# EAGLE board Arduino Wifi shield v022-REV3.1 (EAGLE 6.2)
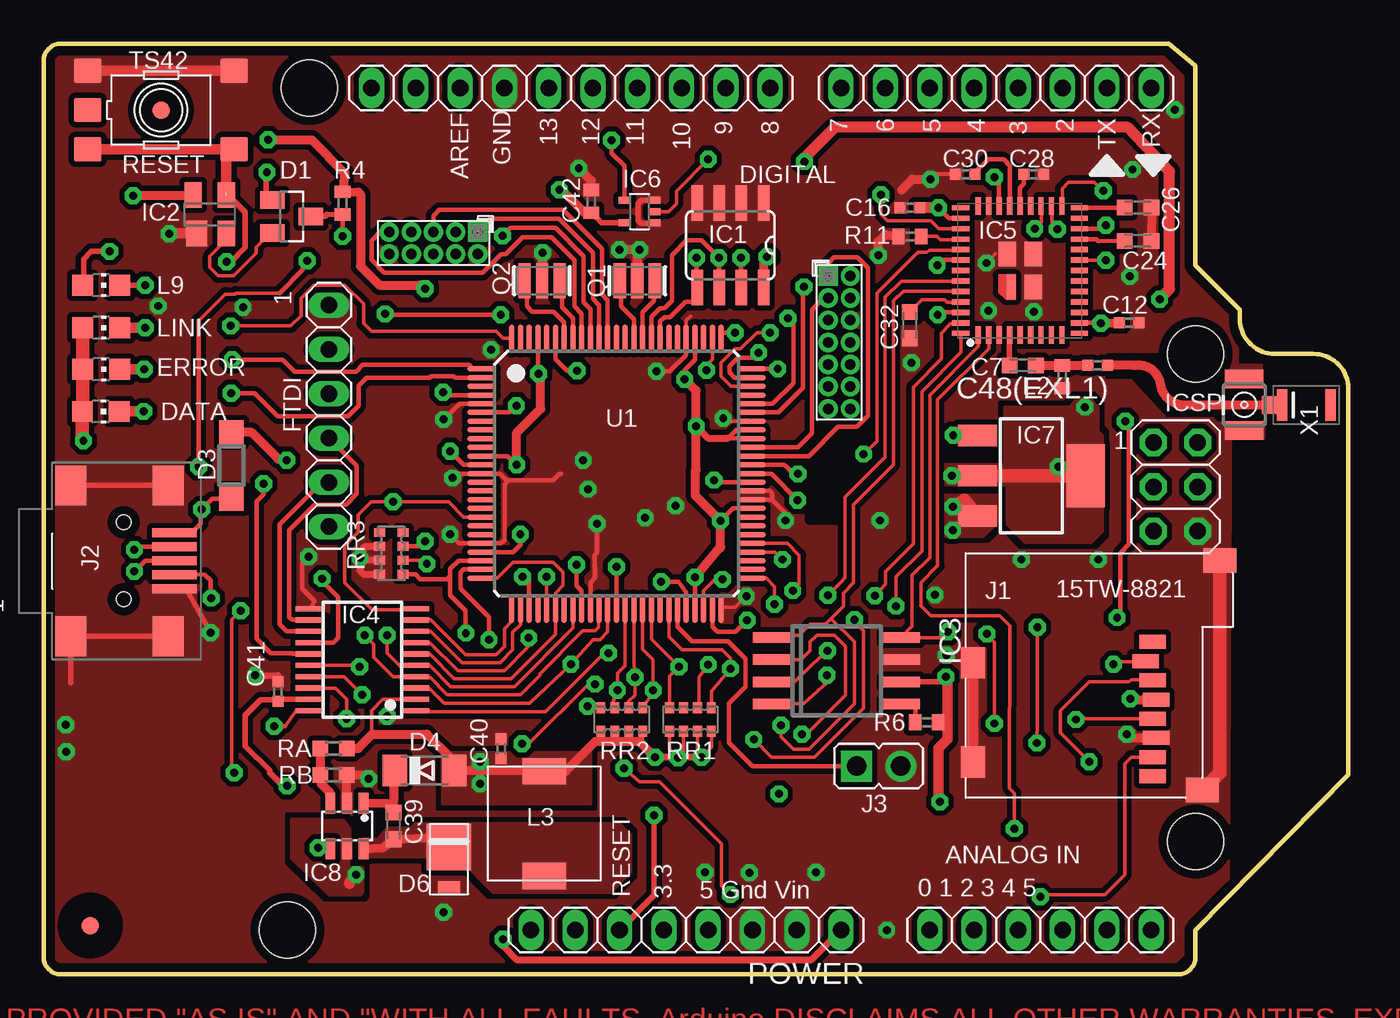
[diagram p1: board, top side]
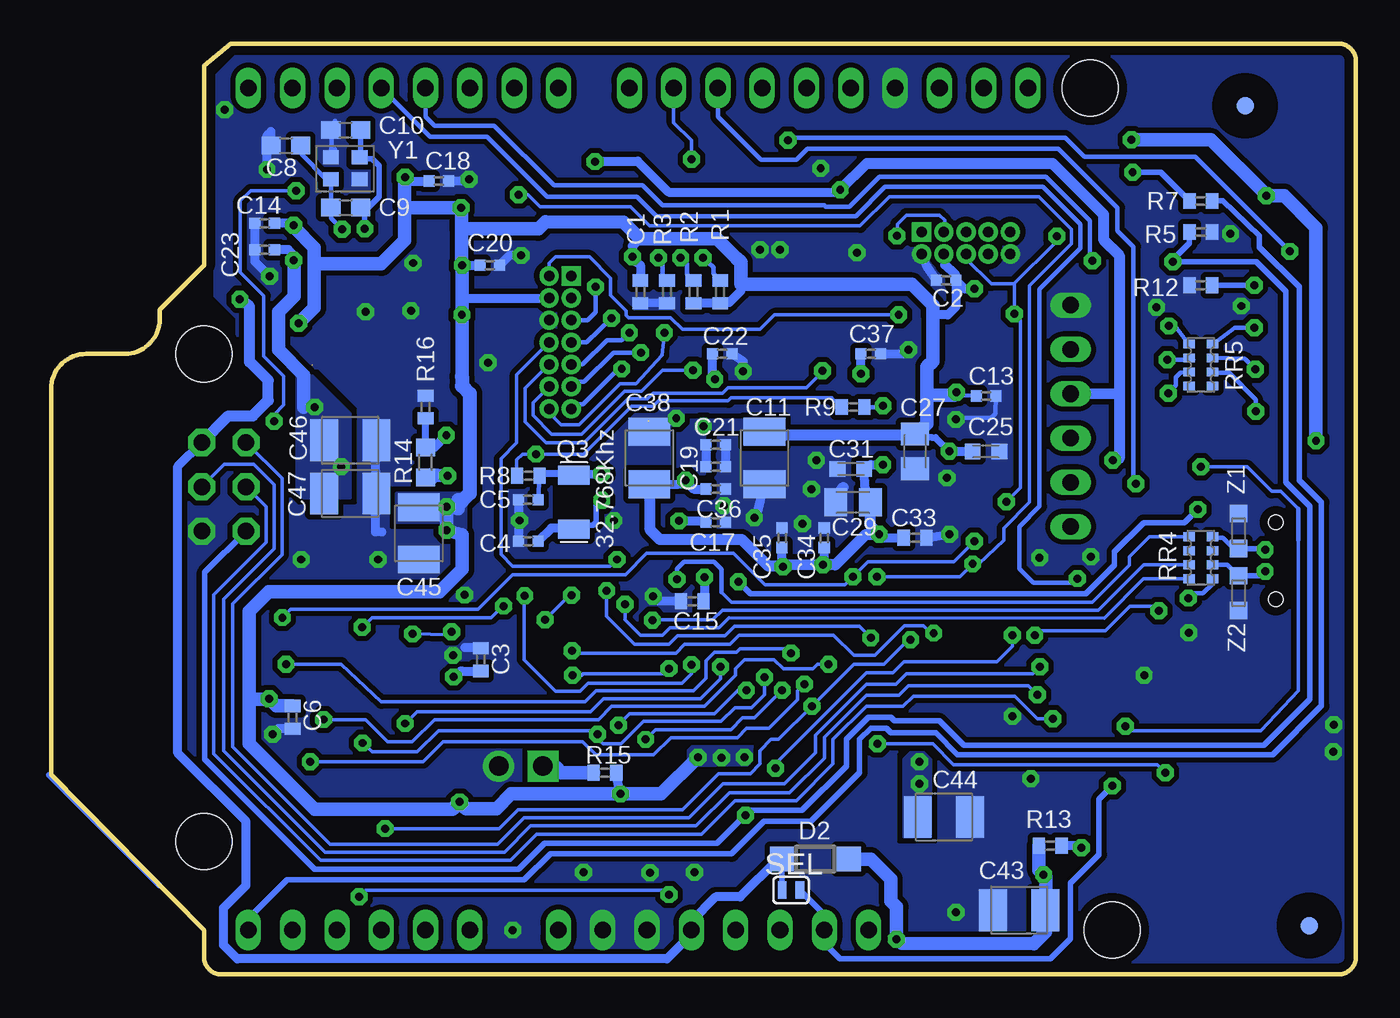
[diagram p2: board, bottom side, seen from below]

Size 74.8 x 53.34 mm. Coordinates in mm from the lower left corner, seen from the top.
Outline: 64.52,53.34 66.04,52.07 66.04,40.64 68.58,38.1 68.58,37.56 arc90 70.58,35.56 72.8,35.56 arc-90 74.8,33.56 74.8,11.43 66.04,2.54 66.04,1 arc-90 65.04,0 1,0 arc-90 0,1 0,52.34 arc-90 1,53.34 64.52,53.34
Copper layers (1*16): Top 0.035mm / dielectric 1.5mm / Bottom 0.035mm
Design rules "default": minimum track width 8mil, minimum drill 16mil, track to track 9mil, track to pad 9mil, pad to pad 9mil, via to via 9mil, smd to smd 7mil, copper to edge 20mil, drill to drill 12mil, minimum pad ring 10mil, minimum via ring 10mil, stop-mask expansion 2mil, vias tented up to drill 24mil, thermal gap 10mil
Net classes: 0 default: width 0.203 mm, drill 0.305 mm, clearance 0.178 mm; 1 power: width 0.254 mm, drill 0.61 mm, clearance 0.203 mm; 2 VIN: width 0.61 mm, drill 0.813 mm, clearance 0.305 mm; 3 usbvcc: width 0.508 mm, drill 0.508 mm, clearance 0.152 mm; 4 aref: width 0.406 mm
Holes 3.2 mm at 66.04,35.56 66.04,7.62 15.24,50.8 13.97,2.54

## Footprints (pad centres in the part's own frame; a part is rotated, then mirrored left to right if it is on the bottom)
1X06-TH = drill 0.95 pad 1.422 long: 1 -6.35,0; 2 -3.81,0; 3 -1.27,0; 4 1.27,0; 5 3.81,0; 6 6.35,0
C0402 = smd 0.7 x 0.9: 1 -0.65,0; 2 0.65,0
C0402' = smd 0.635 x 0.635: 1 -0.559,0; 2 0.559,0
C0603K = smd 0.889 x 0.889: 1 -0.762,0 | smd 0.912 x 0.889: 2 0.762,0
C0603 = smd 1.1 x 1: 1 -0.85,0; 2 0.85,0
SMC_B = smd 1.6 x 2.4: + -1.5,0; - 1.5,0
C0805K = smd 1.3 x 1.6: 1 -1,0; 2 1,0
SOT23 = smd 1 x 1.4: 1 -0.95,-1.1; 2 0.95,-1.1; 3 0,1.1
DIODE_SOD123 = smd 1.4 x 1.4: A 1.9,0; C -1.9,0
MINIMELF = smd 1.4 x 1.8: A 1.7,0; C -1.7,0
DO220AAL = smd 2.667 x 2.54: P$1 -0.7,0 | smd 0.762 x 1.27: P$2 1.65,0
CHIP-LED0805 = smd 1.2 x 1.2: A 0,-1.05; C 0,1.05
1X08-TH = drill 0.95 pad 1.422 long: 1 -8.89,0; 2 -6.35,0; 3 -3.81,0; 4 -1.27,0; 5 1.27,0; 6 3.81,0; 7 6.35,0; 8 8.89,0
1X10-TH = drill 0.95 pad 1.422 long: 1 -11.43,0; 2 -8.89,0; 3 -6.35,0; 4 -3.81,0; 5 -1.27,0; 6 1.27,0; 7 3.81,0; 8 6.35,0; 9 8.89,0; 10 11.43,0
SO08 = smd 0.66 x 2.032: 1 -1.905,-2.413; 2 -0.635,-2.413; 3 0.635,-2.413; 4 1.905,-2.413; 5 1.905,2.413; 6 0.635,2.413; 7 -0.635,2.413; 8 -1.905,2.413
ARDUINO_WIFI_SOT143 = smd 1.2 x 1.44: 1 -0.75,-1.1 | smd 1 x 1.44: 2 0.95,-1.1; 3 0.95,1.1; 4 -0.95,1.1
8S2 = smd 0.6 x 2.2: P$1 -1.905,-3.683; P$2 -0.635,-3.683; P$3 0.635,-3.683; P$4 1.905,-3.683; P$5 1.905,3.683; P$6 0.635,3.683; P$7 -0.635,3.683; P$8 -1.905,3.683
TSSOP20 = smd 0.3 x 1.651: 1 -2.925,-3; 2 -2.275,-3; 3 -1.625,-3; 4 -0.975,-3; 5 -0.325,-3; 6 0.325,-3; 7 0.975,-3; 8 1.625,-3; 9 2.275,-3; 10 2.925,-3; 11 2.925,3; 12 2.275,3; 13 1.625,3; 14 0.975,3; 15 0.325,3; 16 -0.325,3; 17 -0.975,3; 18 -1.625,3; 19 -2.275,3; 20 -2.925,3
QFN-44-7X7 = smd 0.3 x 1: 1 -2.4,-3.7; 2 -1.8,-3.7; 3 -1.2,-3.7; 4 -0.6,-3.7; 5 0,-3.7; 6 0.6,-3.7; 7 1.2,-3.7; 8 1.8,-3.7; 9 2.4,-3.7; 23 2.4,3.7; 24 1.8,3.7; 25 1.2,3.7; 26 0.6,3.7; 27 0,3.7; 28 -0.6,3.7; 29 -1.2,3.7; 30 -1.8,3.7; 31 -2.4,3.7 | smd 1 x 0.3: 10 3.4,-3.6; 11 3.4,-3; 12 3.4,-2.4; 13 3.4,-1.8; 14 3.4,-1.2; 15 3.4,-0.6; 16 3.4,0; 17 3.4,0.6; 18 3.4,1.2; 19 3.4,1.8; 20 3.4,2.4; 21 3.4,3; 22 3.4,3.6; 32 -3.4,3.6; 33 -3.4,3; 34 -3.4,2.4; 35 -3.4,1.8; 36 -3.4,1.2; 37 -3.4,0.6; 38 -3.4,0; 39 -3.4,-0.6; 40 -3.4,-1.2; 41 -3.4,-1.8; 42 -3.4,-2.4; 43 -3.4,-3; 44 -3.4,-3.6 | smd 0.5 x 1.4: 45 -0.5,-0.95 | smd 1 x 1.4: 46 0.75,-0.95; 47 0.75,0.95; 48 -0.75,0.95
SC70-5 = smd 0.4 x 0.7: 1 -0.65,-0.85; 2 0,-0.85; 3 0.65,-0.85; 4 0.65,0.85; 5 -0.65,0.85
SOT223 = smd 1.219 x 2.235: 1 -2.311,-3.099; 2 0,-3.099; 3 2.311,-3.099 | smd 3.6 x 2.2: 4 0,3.099
SOT23-6L = smd 0.55 x 1.2: 1 -0.95,-1.3; 2 0,-1.3; 3 0.95,-1.3; 4 0.95,1.3; 5 0,1.3; 6 -0.95,1.3
2X03 = drill 0.95 pad 1.55 octagon: 1 -2.54,-1.27; 2 -2.54,1.27; 3 0,-1.27; 4 0,1.27; 5 2.54,-1.27; 6 2.54,1.27
SDCARD-15TW-8821 = smd 0.8 x 1.5: 1 0,0; 2 1.1,-0.4; 3 2.2,0; 4 3.3,0.2; 5 4.4,0; 6 5.5,0.2; 7 6.6,0; 8 7.7,0 | smd 1.4 x 1.9: SH1 -4.66,3.85; SH2 8.49,2.85 | smd 1.8 x 1.4: SH3 1.19,-10.3; SH4 6.89,-10.3
USB-MINI-B_2 = smd 0.508 x 2.54: 1 0,0; 2 0.8,0; 3 1.6,0; 4 2.4,0; 5 3.2,0 | smd 2.286 x 1.778: 6 -2.717,5.948; 7 -2.717,0.36; 8 5.918,0.36; 9 5.918,5.948 | hole 0.813: -0.6,2.9; 3.8,2.9
JP1 = drill 1.118 pad 1.778 square: 1 0,-1.27 | drill 1.118 pad 1.778: 2 0,1.27
PINHEAD_2X05_127 = drill 0.6 pad 1.016 square: 1 -0.635,2.54 | drill 0.6 pad 1.016: 2 0.635,2.54; 3 -0.635,1.27; 4 0.635,1.27; 5 -0.635,0; 6 0.635,0; 7 -0.635,-1.27; 8 0.635,-1.27; 9 -0.635,-2.54; 10 0.635,-2.54
L0402 = smd 0.7 x 0.9: 1 -0.65,0; 2 0.65,0
SRR0604 = smd 1.5 x 2.5: P$1 3,0; P$2 -3,0
PINHEAD_2X07_127 = drill 0.6 pad 1.016 square: 1 -0.635,3.81 | drill 0.6 pad 1.016: 2 0.635,3.81; 3 -0.635,2.54; 4 0.635,2.54; 5 -0.635,1.27; 6 0.635,1.27; 7 -0.635,0; 8 0.635,0; 9 -0.635,-1.27; 10 0.635,-1.27; 11 -0.635,-2.54; 12 0.635,-2.54; 13 -0.635,-3.81; 14 0.635,-3.81
SMD_RESONATOR = smd 0.7 x 2: 1 -1,0; 2 0,0; 3 1,0
RESONATOR_EPSON_FC_145 = smd 1.1 x 1.8: P$1 -1.55,0; P$2 1.55,0
R0402 = smd 0.7 x 0.9: 1 -0.65,0; 2 0.65,0
R0603 = smd 1 x 1.1: 1 -0.85,0; 2 0.85,0
R0603' = smd 0.889 x 0.889: 1 -0.762,0; 2 0.762,0
ST-MOD_V1.4_TS42 = smd 1.6 x 1.4: 1 -4.2,2.25; 2 4.2,2.25; 3 -4.2,-2.25; 4 4.2,-2.25; 5 -4.2,0
CAY16 = smd 0.5 x 0.65: 1 -1.2,-0.675; 2 -0.4,-0.675; 3 0.4,-0.675; 4 1.2,-0.675; 5 1.2,0.675; 6 0.4,0.675; 7 -0.4,0.675; 8 -1.2,0.675
SJL = smd 0.508 x 1.016: 1 -0.508,0; 2 0.508,0
TQFP100 = smd 1.6 x 0.305: 1 -7.747,6; 2 -7.747,5.5; 3 -7.747,5; 4 -7.747,4.5; 5 -7.747,4; 6 -7.747,3.5; 7 -7.747,3; 8 -7.747,2.5; 9 -7.747,2; 10 -7.747,1.5; 11 -7.747,1; 12 -7.747,0.5; 13 -7.747,0; 14 -7.747,-0.5; 15 -7.747,-1; 16 -7.747,-1.5; 17 -7.747,-2; 18 -7.747,-2.5; 19 -7.747,-3; 20 -7.747,-3.5; 21 -7.747,-4; 22 -7.747,-4.5; 23 -7.747,-5; 24 -7.747,-5.5; 25 -7.747,-6; 51 7.747,-6; 52 7.747,-5.5; 53 7.747,-5; 54 7.747,-4.5; 55 7.747,-4; 56 7.747,-3.5; 57 7.747,-3; 58 7.747,-2.5; 59 7.747,-2; 60 7.747,-1.5; 61 7.747,-1; 62 7.747,-0.5; 63 7.747,0; 64 7.747,0.5; 65 7.747,1; 66 7.747,1.5; 67 7.747,2; 68 7.747,2.5; 69 7.747,3; 70 7.747,3.5; 71 7.747,4; 72 7.747,4.5; 73 7.747,5; 74 7.747,5.5; 75 7.747,6 | smd 0.305 x 1.6: 26 -6,-7.747; 27 -5.5,-7.747; 28 -5,-7.747; 29 -4.5,-7.747; 30 -4,-7.747; 31 -3.5,-7.747; 32 -3,-7.747; 33 -2.5,-7.747; 34 -2,-7.747; 35 -1.5,-7.747; 36 -1,-7.747; 37 -0.5,-7.747; 38 0,-7.747; 39 0.5,-7.747; 40 1,-7.747; 41 1.5,-7.747; 42 2,-7.747; 43 2.5,-7.747; 44 3,-7.747; 45 3.5,-7.747; 46 4,-7.747; 47 4.5,-7.747; 48 5,-7.747; 49 5.5,-7.747; 50 6,-7.747; 76 6,7.747; 77 5.5,7.747; 78 5,7.747; 79 4.5,7.747; 80 4,7.747; 81 3.5,7.747; 82 3,7.747; 83 2.5,7.747; 84 2,7.747; 85 1.5,7.747; 86 1,7.747; 87 0.5,7.747; 88 0,7.747; 89 -0.5,7.747; 90 -1,7.747; 91 -1.5,7.747; 92 -2,7.747; 93 -2.5,7.747; 94 -3,7.747; 95 -3.5,7.747; 96 -4,7.747; 97 -4.5,7.747; 98 -5,7.747; 99 -5.5,7.747 | smd 0.3 x 1.6: 100 -6,7.747
FIDUCIA-MOUNT = smd 1.016 x 1.016: P$1 0,0
LDA31 = smd 1.8 x 0.6: 1 0,-1.4; 2 0,1.4
MC-921 = smd 1 x 1.05: 1 0,1.528 | smd 1.05 x 2.2: 2@1 -1.475,0; 2@2 1.475,0
ARDUINO_WIFI_2.5X2.0 = smd 0.9 x 0.8: 1 -0.85,-0.65; 2 0.8,-0.65; 3 0.8,0.6; 4 -0.85,0.6
CT/CN0603 = smd 1 x 1: 1 -1,0; 2 1,0

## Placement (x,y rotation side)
ANALOG_IN  [1X06-TH]  57.15,2.54 0 top
C1  0.1uF  [C0402]  41.02,39.12 270 bottom
C2  0.1uF  [C0402']  23.5,39.78 180 bottom
C3  0.1uF  [C0402]  50.16,18.03 90 bottom
C4  22pF  [C0402']  47.45,24.82 0 bottom
C5  22pF  [C0402']  47.45,27.2 0 bottom
C6  0.1uF  [C0402]  60.96,14.73 270 bottom
C7  1pF  [C0603K]  56.13,34.9 0 top
C8  N.M.  [C0603]  61.34,47.5 0 bottom
C9  0.5pF_NM  [C0603]  57.91,43.94 0 bottom
C10  N.M.  [C0603]  57.91,48.39 0 bottom
C11  10uF  [SMC_B]  33.91,29.59 270 bottom
C12  1uF  [C0402']  62.23,37.34 0 top
C13  1uF  [C0402']  21.21,33.15 0 bottom
C14  1uF  [C0402']  62.56,43.05 180 bottom
C15  1uF  [C0402]  38.05,21.39 180 bottom
C16  1uF  [C0402']  49.66,43.94 180 top
C17  1uF  [C0402']  36.7,25.91 0 bottom
C18  0.1uF  [C0402']  52.58,45.47 0 bottom
C19  1uF  [C0402']  36.7,29.08 0 bottom
C20  0.1uF  [C0402']  49.66,40.64 0 bottom
C21  1uF  [C0402']  36.7,30.35 0 bottom
C22  1uF  [C0402']  36.32,35.56 0 bottom
C23  1uF  [C0402']  62.56,41.53 180 bottom
C24  22pF  [C0603K]  62.74,42.04 0 top
C25  2.2nF (1nF)  [C0603K]  21.21,29.97 0 bottom
C26  22pF  [C0603K]  62.74,43.94 0 top
C27  2.2uF(4.7uF)  [C0805K]  25.27,29.97 270 bottom
C28  0.1uF  [C0402']  56.77,45.85 0 top
C29  2.2uF  [C0805K]  28.83,27.05 180 bottom
C30  1uF  [C0402']  52.83,45.85 180 top
C31  2.2nF (470pF)  [C0603K]  28.96,28.96 180 bottom
C32  0.33uF  [C0603K]  49.66,37.21 270 top
C33  1uF  [C0402]  25.27,25.02 0 bottom
C34  1uF  [C0402']  30.48,25.02 90 bottom
C35  1uF  [C0402']  32.89,25.02 90 bottom
C36  1uF  [C0402']  36.7,27.81 0 bottom
C37  1uF  [C0402']  27.81,35.56 0 bottom
C38  10uF  [SMC_B]  40.51,29.59 90 bottom
C39  10nF  [C0603K]  20.07,8.51 270 top
C40  0.1uF  [C0402']  26.24,12.93 90 top
C41  0.1uF  [C0402']  13.44,16.21 90 top
C42  0.1uF  [C0402]  31.39,44.3 90 top
C43  10uF  [SMC_B]  19.3,3.68 180 bottom
C44  10uF  [SMC_B]  23.62,9.02 0 bottom
C45  10uF  [SMC_B]  53.72,25.27 270 bottom
C46  10uF  [SMC_B]  57.66,30.61 0 bottom
C47  10uF  [SMC_B]  57.66,27.56 0 bottom
C48(EXL1)  0.5pF  [C0402']  60.43,34.9 180 top
D1  BAT54A  [SOT23]  14.22,43.43 270 top
D2  MBR0520  [DIODE_SOD123]  30.99,6.6 180 bottom
D3  MBR0520  [DIODE_SOD123]  10.77,29.16 270 top
D4  CD1206-S01575  [MINIMELF]  21.84,11.68 0 top
D6  SS1P3L  [DO220AAL]  23.24,6.6 270 top
DATA  Blue  [CHIP-LED0805]  3.28,32.26 270 top
DIGITAL_1  [1X08-TH]  54.61,50.8 180 top
DIGITAL_2  [1X10-TH]  30.23,50.8 180 top
ERROR  Red  [CHIP-LED0805]  3.3,34.67 270 top
FTDI  [1X06-TH]  16.36,32 270 top
IC1  AT24C128BN-SH-B  [SO08]  39.37,41.78 180 top
IC2  ADM811  [ARDUINO_WIFI_SOT143]  9.53,43.56 0 top
IC3  AT45DB021D-SH-B  [8S2]  45.47,17.4 270 top
IC4  TXB0108  [TSSOP20]  18.29,18.03 90 top
IC5  HDG104  [QFN-44-7X7]  55.98,40.34 0 top
IC6  74LVC1G125  [SC70-5]  34.16,43.71 90 top
IC7  LM1117-ADJ  [SOT223]  56.64,28.57 270 top
IC8  LM2736  [SOT23-6L]  17.4,8.51 180 top
ICSP  [2X03]  64.9,27.94 270 top
J1  15TW-8821  [SDCARD-15TW-8821]  63.58,19.05 270 top
J2  5075BMR-05-SM  [USB-MINI-B_2]  7.49,22.1 90 top
J3  [JP1]  47.88,11.94 270 top
JTAG  [PINHEAD_2X05_127]  22.35,41.91 270 top
L2  3.9nH  [L0402]  58.39,34.24 90 top
L3  10u SRR0604-100ML  [SRR0604]  28.7,8.64 270 top
L9  Yellow  [CHIP-LED0805]  3.3,39.5 270 top
LINK  Green  [CHIP-LED0805]  3.3,37.06 270 top
MACB  [PINHEAD_2X07_127]  45.62,36.22 0 top
POWER  [1X08-TH]  36.83,2.54 180 top
Q1  12MHz  [SMD_RESONATOR]  34.04,39.75 180 top
Q2  N.M.  [SMD_RESONATOR]  28.57,39.75 180 top
Q3  32.768Khz  [RESONATOR_EPSON_FC_145]  44.83,27.05 270 bottom
R1  10K  [R0402]  36.45,39.12 90 bottom
R2  10K  [R0402]  37.97,39.12 90 bottom
R3  10K  [R0402]  39.5,39.12 270 bottom
R4  100K  [R0402]  17.14,44.2 270 top
R5  100K  [R0402]  8.89,42.55 180 bottom
R6  10K  [R0402]  50.62,14.45 0 top
R7  N.M.  [R0402]  8.89,44.32 180 bottom
R8  N.M.  [R0402]  47.45,28.57 180 bottom
R9  0R  [R0402]  28.83,32.51 180 bottom
R11  100K  [R0402]  49.66,42.29 180 top
R12  1K  [R0402]  8.89,39.5 180 bottom
R13  100K  [R0402]  17.53,7.37 180 bottom
R14  1K  [R0603]  53.34,29.34 270 bottom
R15  10K  [R0402]  43.05,11.56 180 bottom
R16  0R  [R0402]  53.34,32.51 270 bottom
RA  16.5K  [R0603']  16.64,12.95 180 top
RB  10K  [R0603']  16.64,11.43 180 top
RESET  TS42  [ST-MOD_V1.4_TS42]  6.73,49.53 0 top
RR1  10K/100K  [CAY16]  37.08,14.61 180 top
RR2  10K/100K  [CAY16]  33.15,14.61 180 top
RR3  10K  [CAY16]  19.94,24.13 270 top
RR4  22R  [CAY16]  8.89,23.88 270 bottom
RR5  1K  [CAY16]  8.89,34.92 270 bottom
SEL  NM  [SJL]  32.38,4.83 0 bottom
U1  AT32UC3A1256(512)  [TQFP100]  32.84,28.7 0 top
U$1  FIDUCIALMOUNT  [FIDUCIA-MOUNT]  6.73,49.53 0 top
U$2  FIDUCIALMOUNT  [FIDUCIA-MOUNT]  2.67,2.79 0 top
U$3  FIDUCIALMOUNT  [FIDUCIA-MOUNT]  2.67,2.79 0 bottom
U$4  FIDUCIALMOUNT  [FIDUCIA-MOUNT]  6.35,49.78 0 bottom
U$5  DISCLAIMER  [DISCLAIMER]  not placed on the board
X1  LDA312G7313F-237  [LDA31]  72.39,32.64 270 top
X4  MC-921_NM  [MC-921]  68.83,32.64 270 top
Y1  40MHz 8pF  [ARDUINO_WIFI_2.5X2.0]  57.91,46.23 0 bottom
Z1  CG0603MLC-05E  [CT/CN0603]  6.73,25.4 270 bottom
Z2  CG0603MLC-05E  [CT/CN0603]  6.73,21.84 90 bottom

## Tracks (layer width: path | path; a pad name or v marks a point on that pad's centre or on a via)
!RESET_3V3  (via drill 0.46)
  Top 0.203: U1.18 24.09,26.2 23.22,27.08 v20.04,27.08 18.77,27.08 18.03,26.34 18.03,25.32 17.27,24.56 17.27,22.45 18.82,20.9 21.54,20.9 IC4.10
  Top 0.254: v17.14,42.29 R4.2 | v26.21,37.8 19.63,37.8 v19.58,37.85
  Top 0.305: R4.2 16.26,43.56 16.13,43.43 D1.3
  Bottom 0.203: v17.14,42.29 17.27,41.91 19.58,39.6 | JTAG.6 22.35,41.02 20.9,39.57 19.61,39.57 19.58,39.6 | v19.58,37.85 19.58,39.6 | 19.47,37.73 19.23,37.49 19.23,27.89 v20.04,27.08 | MACB.2 46.25,40.74 45.87,41.12 43.94,41.12 42.72,39.9 42.72,38.91 41.83,38.02 41.83,37.77 41.71,37.64 39.29,37.64 38.61,36.96 34.16,36.96 33.33,37.8 v26.21,37.8
  Bottom 0.254: 19.47,37.73 v19.58,37.85
+1V2  (via drill 0.46)
  Top 0.203: IC5.17 60.89,40.94 v60.91,40.92
  Top 0.762: IC7.4 IC7.2 v52.07,28.57
  Bottom 0.508: v60.91,40.92 60.91,41.22 61.21,41.53 C23.1
  Bottom 0.762: v52.07,28.57 52.2,28.57 53.03,28.63 52.92,28.5 R14.2 | 60.33,32.51 60.33,34.34 61.77,35.79 61.77,37.97 60.88,38.86 60.88,40.89 v60.91,40.92
  other vias: 59.69,32.51 58.17,29.08
  pour Bottom (isolate 0.305, no thermals): 57.66,27.3 57.66,32.13 59.82,34.29 60.71,34.29 60.71,27.69 60.33,27.3
  pour Top (isolate 0.305, no thermals): 51.69,29.21 55.12,29.21 55.12,32.51 58.8,32.51 59.31,33.02 59.94,33.02 60.45,32.51 60.45,31.11 60.71,30.86 60.71,25.4 60.07,24.77 56.26,24.77 55.24,25.78 55.24,28.07 51.69,28.07
+1V8  (via drill 0.46)
  Top 0.254: v38.44,28.33 38.48,28.19 38.74,28.2 U1.62 | U1.22 26.92,24.2 27.33,24.61 v27.33,25.22 | v30.56,23.47 30.56,22.28 30.84,22 U1.34 | v32.84,23.37 U1.38 | U1.97 28.34,34.45 v28.37,34.42 | U1.11 26.6,29.7 v27.13,29.21
  Top 0.508: v27.13,29.21 27.13,31.04 28.5,32.41 28.5,34.29 v28.37,34.42
  Bottom 0.203: v38.44,28.33 38.61,27.94 39.37,27.94 C38.+
  Bottom 0.508: v27.33,25.22 27.13,25.02 C33.1 | v28.37,34.42 C37.1 | v38.44,28.33 38.4,28.2 37.97,27.81 C36.1 | C38.+ 38.84,28.09 | C35.1 32.89,23.44 32.84,23.39 32.82,23.39 v32.84,23.37 | v30.56,23.47 30.48,23.39 C34.1 | C29.1 28.08,27.32 C31.1 27.81,29.21 v27.13,29.21
  Bottom 0.61: v30.56,23.47 32.74,23.47 v32.84,23.37
  Bottom 0.635: C29.1 27.83,25.72 v27.33,25.22 27.36,25.2 28.12,25.2 29.84,23.47 v30.56,23.47 | v32.84,23.37 32.82,23.34 | 32.82,23.39 33.68,23.39 35.2,24.92 39.9,24.92 40.46,25.48 40.46,28.12 C38.+
+3V3  (via drill 0.46)
  Top 0.203: IC4.2 19.44,15.76 18.8,15.11 18.8,13.82 18.85,13.77 | RR2.5 31.95,13.27 32.13,13.34 | RR2.6 32.75,13.23 32.64,13.34 | RR2.7 33.55,13.23 33.4,13.34 | RR2.8 34.35,13.27 34.16,13.34 | RR1.8 38.28,13.01 v37.72,12.45 37.48,12.68 RR1.7 | RR1.6 36.68,12.73 v36.37,12.42 35.88,12.91 RR1.5
  Top 0.254: U1.79 37.34,35.21 36.75,34.62 v36.75,34.11 | U1.59 39.53,26.7 v38.81,25.98 | U1.12 24.09,29.2 v23.32,29.97 | U1.4 23.06,33.2 v22.91,33.35 | IC5.29 54.78,45.52 v54.51,45.7 | IC5.20 60.72,42.73 v60.91,42.93 | U1.47 37.34,23.01 v37.34,22.76 | IC5.37 arc45 52.56,40.95 51.54,40.95 v51.23,40.64 | IC5.11 60.58,37.34 v60.6,37.31 | IC5.33 51.91,43.34 v51.31,43.94 | IC5.42 51.4,37.94 v51.26,37.8 | v51.74,17.04 51.46,16.76 | U1.67 40.56,30.73 39.24,30.73 39.71,31.2 U1.68
  Top 0.305: 51.46,16.76 IC3.P$6
  Top 0.406: v37.72,12.45 v35.05,12.45 | v37.41,31.42 38.1,30.73 39.24,30.73
  Top 0.508: v21.87,39.29 21.59,39.5 19.25,39.5 18.16,40.59 18.16,44.7 18.03,44.83 R4.1 17.27,45.92 15.37,47.83 v12.88,47.83 | 29.27,11.68 D4.A 23.24,11.99 23.24,12.5 21.97,13.77 18.85,13.77 18.03,12.95 RA.1 | 38.76,24.43 38.79,24.43 | v37.34,22.76 38.76,24.43 | IC2.4 5.16,44.66 v5.13,44.63 | J1.4 62.48,15.75 v62.31,15.8 | v60.6,37.31 C12.1 | IC1.8 41.27,40.79 v41.48,41.12 | 38.76,24.43 38.81,24.49 v38.81,25.98 37.36,27.43 37.36,28.85 37.41,28.91 v37.41,31.42 37.41,33.45 v36.75,34.11 | L3.P$2 29.92,11.64 31.62,13.34 32.13,13.34 32.64,13.34 33.4,13.34 34.16,13.34 v35.05,12.45
  Top 0.61: v51.74,17.04 51.82,17.04 51.82,14.48 | 51.82,14.48 51.82,13.46 51.31,12.95 51.31,9.96 v51.38,9.88 | R6.2 51.79,14.45 51.82,14.48 | D4.A 23.29,11.94
  Top 0.635: v51.31,43.94 C16.1
  Top 0.762: LINK.A ERROR.A 2.25,32.28 DATA.A 2.23,30.64 v2.29,30.58 | IC7.3 52.78,27.18 v52.12,26.8
  Bottom 0.254: 51.28,42.72 51.28,43.92 v51.31,43.94 | v22.91,33.35 22.66,33.35 22.5,33.2 C13.1
  Bottom 0.406: 25.15,30.89 24.11,30.76 v23.32,29.97
  Bottom 0.508: v23.32,29.97 C25.1 | C21.1 C19.1 | C22.1 36.88,34.19 v36.75,34.11 | v60.91,42.93 61.04,43.05 C14.1 | v37.34,22.76 37.34,21.45 C15.1 | C3.1 51.26,17.37 51.31,17.37 51.64,17.04 v51.74,17.04 | 62.28,15.77 v62.31,15.8 | R15.1 42.18,10.35 v42.16,10.34 | v51.23,40.64 C20.1 | MACB.4 51,38.76 51.23,38.99 | C1.1 41.02,40.64 41.27,40.82 v41.48,41.12 41.48,41.73 41.05,42.16 | R2.1 R1.1 36.45,38.51 35.92,38.51 35.26,39.17 35.26,39.55 | C2.1 22.4,39.27 v21.87,39.29 | C2.1 22.94,38.25 23.39,37.8 24.26,37.8 | C18.1 54.28,45.47 v54.51,45.7 | C17.1 37.69,25.98 v38.81,25.98 | C2.1 22.94,40.08 22.99,40.13 23.57,40.66 JTAG.4
  Bottom 0.635: C27.1 25.04,30.84 25.15,30.89 33.73,30.89 C11.+
  Bottom 0.762: v12.88,47.83 8.31,47.83 5.26,44.78 v5.13,44.63 4.12,44.63 3.12,43.64 3.12,43.61 2.29,42.77 v2.29,30.58 | 51.49,27.2 51.49,26.7 C45.+ | 51.28,42.72 51.28,40.76 arc-45 v51.23,40.64 51.23,38.99 51.23,37.82 v51.26,37.8 51.26,34.27 | 51.28,42.72 51.28,43.94 v51.31,43.94 54.51,43.94 54.53,43.92 | v42.16,10.34 39.83,10.34 v37.72,12.45 | 42.18,10.35 48.42,10.35 49.28,9.5 51,9.5 v51.38,9.88 51.79,9.47 59.69,9.47 63.45,13.21 63.45,15.77 | C6.1 61.89,15.38 62.28,15.77 63.45,15.77 | 63.45,15.77 63.45,20.8 62.33,21.92 52.53,21.92 51.23,23.22 51.23,25.2 v52.12,25.45 v52.12,26.8 | 54.53,43.92 54.53,42.06 55.88,40.72 59.72,40.72 | 59.72,40.72 59.72,41.63 60.83,42.8 60.88,42.85 60.88,42.93 v60.91,42.93 | 59.72,40.72 59.72,40.23 59.71,38.2 60.58,37.34 v60.6,37.31 | 54.53,43.92 54.53,45.72 v54.51,45.7 | 51.28,42.72 46.86,42.72 46.46,43.13 41.99,43.1 41.05,42.16 36.63,42.16 35.53,41.07 35.26,40.82 35.26,39.55 25.45,39.55 24.26,38.35 24.26,37.8 24.26,35.13 24.59,34.82 24.59,33.2 | C27.1 25.09,31.05 24.59,31.55 24.59,33.2 | 24.59,33.2 23.06,33.2 v22.91,33.35
  Bottom 0.813: 51.26,34.27 51.26,33.73 50.8,33.27 50.8,27.56 51.56,26.8 v52.12,26.8
  other vias: 25.02,12.19 25.02,10.92
  pour Top (isolate 0.305, no thermals): 22.86,12.7 22.86,9.78 31.37,9.78 31.37,12.7
  pour Bottom (isolate 0.305, no thermals): 25.02,12.7 24.77,12.7 24.38,12.32 24.38,7.87 25.91,7.87 25.91,12.32 25.53,12.7
  pour Bottom (isolate 0.254, no thermals): 53.31,27.43 53.31,27.48 53.29,27.51 52.81,27.51 52.78,27.48
  pour Bottom (isolate 0.254, no thermals): 51.05,27.56 54.99,27.56 54.99,25.91 52.2,25.91 51.82,25.53 51.05,25.53
  pour Bottom (isolate 0.305, no thermals): 34.57,13.03 38.07,13.03 38.25,12.85 38.25,12.14 38.13,11.99 34.77,11.99 34.57,12.19
  pour Bottom (isolate 0.305, no thermals): 33.78,30.48 33.78,31.75 38.86,31.75 38.86,28.7 37.34,28.7 37.34,31.24 34.98,31.24 34.98,30.48
  pour Top (isolate 0.305, no thermals): 54.61,27.43 51.69,27.43 51.69,25.15 53.85,25.15 54.61,25.91
+5V  (via drill 0.46)
  Top 0.305: IC6.5 31.98,43.06 C42.1
  Top 0.508: D3.C 11.92,31.06 13.44,29.55 v13.95,29.46 | C42.1 31,43.65 29.84,44.83 29.72,44.96 v29.57,44.96
  Top 0.635: v63.98,38.68 64.54,39.27 64.54,46.02 62.15,48.54 45.44,48.54 45.34,48.51 43.61,46.79 v43.61,46.58
  Bottom 0.305: SEL.1 D2.A
  Bottom 0.508: v43.61,46.58 43.59,46.61 41.17,46.61 39.4,44.83 29.72,44.83 29.59,44.96 v29.57,44.96 | ICSP.2 67.54,29.11 67.54,12.68 63.63,8.76 63.63,5.11 64.92,3.81 64.92,1.68 64.14,0.89 39.5,0.89 38.1,2.29 POWER.4 38.1,3.05 36.7,4.45 35.31,4.45 33.15,6.6 D2.A
  Bottom 0.61: FTDI.3 13.69,33.27 13.56,33.15 | 27.94,46.48 28.04,46.48 v29.57,44.96
  Bottom 0.635: v63.98,38.68 63.96,38.68 63.42,38.28 63.42,35.1 62.36,34.04 62.36,32.89 63.25,32 64.64,32 ICSP.2 | 27.94,46.48 17.4,46.48 14.48,43.56 14.48,42.11 13.56,41.2 13.56,33.15 13.56,29.57 13.82,29.57 v13.95,29.46
D+  (via drill 0.46)
  Top 0.254: 7.44,23.7 J2.3 | 7.44,23.7 | 7.44,23.7 5.82,23.7 v5.21,23.09
  Bottom 0.254: 8.11,23.48 7.36,23.48 Z2.2
  Bottom 0.305: v5.21,23.09 5.45,22.84 Z2.2 6.75,22.86 | 8.11,23.48 RR4.6
D-  (via drill 0.46)
  Top 0.254: J2.4 5.37,24.5 v5.21,24.33
  Bottom 0.254: RR4.8 8.16,25.02 7.62,25.02 7,24.4 Z1.2
  Bottom 0.305: v5.21,24.33 5.27,24.4 Z1.2 6.75,24.38
DF_CS  (via drill 0.46)
  Top 0.203: U1.44 35.84,19.35 36.6,18.59 38.89,18.59 39.37,18.11 v39.37,17.53 38.28,16.24 RR1.1 | v44.91,17.14 44.91,16.71 43.56,15.49 IC3.P$4
  Bottom 0.203: v44.91,17.14 44.37,17.14 44.3,17.22 39.67,17.22 v39.37,17.53
DF_RESET  (via drill 0.46)
  Top 0.203: v44.93,18.54 44.07,17.78 43.05,16.76 IC3.P$3
  Top 0.254: RR3.5 21.32,22.93 21.59,22.66 23.14,22.66 | 23.14,22.66 23.32,22.66 | U1.23 23.78,23.7 23.32,23.24 23.32,22.84 | 23.32,22.84 23.32,21.72 24.21,20.83 v24.21,19.56 | 23.32,22.84 23.14,22.66
  Bottom 0.203: v44.93,18.54 44.83,18.41 38.99,18.41 38.48,18.92 35.89,18.92 35.38,19.43 29.95,19.43 28.78,18.29 27.57,18.29 25.87,19.99 24.79,19.99 24.49,19.68 v24.21,19.56
EE_SCL  (via drill 0.46)
  Top 0.254: IC1.6 v38.71,41.07 37.72,42.06 36.85,42.06 36.02,41.22 36.02,38.61 35.59,38.18 35.33,38.18 34.84,37.69 U1.84
  Bottom 0.254: v38.71,41.07 38.35,40.72 38.35,40.13 R2.2
EE_SDA  (via drill 0.46)
  Top 0.254: U1.83 35.34,37.42 35.59,37.67 35.92,37.67 36.8,38.56 37.41,38.56 37.47,38.61 IC1.5 v37.44,41.07
  Bottom 0.254: v37.44,41.07 36.83,40.51 36.83,40.15 R1.2
GND  (via drill 0.46)  (1 unrouted)
  Top 0.203: 54.08,40.79 54.57,41.28 | U1.50 38.84,21.03 39.65,21.03 v40.28,21.67 | U1.80 36.84,37.48 37.08,37.72 | 40.51,31.7 39.17,31.7 38.86,32
  Top 0.254: 26.67,28.32 26.54,28.32 26.16,28.7 U1.13 23.7,28.7 v23.44,28.45 | 26.67,28.32 29.21,28.32 29.59,28.7 29.67,28.7 | U1.5 23.86,32.7 22.96,31.8 | IC4.11 15.54,21.39 14.83,22.1 14.83,23.57 v15.19,23.93 | U1.35 31.34,22.45 31.62,22.73 31.6,24.03 31.73,24.16 v31.73,25.83 | C30.2 51.16,45.87 v50.85,45.57 | U1.80 36.84,35.5 36.8,35.46 35.89,34.57 v35.13,34.57 | 26.67,28.32 26.42,28.07 26.42,24.89 26.23,24.7 U1.21 23.81,24.7 v23.29,25.22 | v42.55,26.01 42.55,26.42 41.76,27.2 | U1.61 41.64,27.7 41.76,27.58 41.76,27.2 | U1.60 41.76,27.2
  Top 0.305: IC6.3 34.28,44.36 34.09,44.17 34.09,43.23 34.27,43.05 IC6.1 | J2.9 J2.8 | J2.7 J2.6 1.54,16.7 | J2.1 8.18,22.1 v9.58,19.58
  Top 0.406: RR3.2 18.41,24.53 v18.14,23.88 | v18.14,23.88 18.14,23.14 18.34,22.94 RR3.4 | RR3.3 18.28,23.73 v18.14,23.88 | C41.2 13.44,17.12 v12.14,17.14
  Top 0.508: Q2.2 28.6,39.78 v28.6,41.35 | C42.2 31.39,45.49 v30.68,46.2 | C26.2 63.6,43.89 C24.2 | IC8.2 17.35,11.58 RB.1 18.62,11.43 | J1.6 62.32,13.55 v62.1,13.77 | v47.85,41.2 47.85,41.99 48.26,42.39 R11.2 | 49.2,44.96 49.81,45.57 v50.85,45.57 | Q1.2 34.04,41.43 v34.16,41.53 v33.02,41.53
  Top 0.61: RESET.1 RESET.2 10.62,52.06 | IC2.1 7.21,42.46 v7.19,42.44
  Top 0.635: J1.SH4 J1.SH3
  Top 0.762: J1.SH1 67.43,11.56 J1.SH2
  Bottom 0.254: 58.52,47.3 Y1.4 58.71,47.97 58.52,48.16 58.52,48.91 C10.1 | C13.2 20.68,32.13 20.9,31.9 22.84,31.9 v22.94,31.8
  Bottom 0.508: C37.2 25.91,35.56 25.68,35.81 | C21.2 C19.2 | C11.- 34.34,26.31 v34.49,26.16 | C8.1 62.19,48.3 62.43,48.06 62.43,46.23 | C14.2 C23.2 63.12,40.84 v62.28,40.01 | R3.2 41.14,38.48 C1.2 | v40.28,21.67 40.01,21.39 C15.2 | 51.08,18.72 50.26,18.72 C3.2 | 55.83,25.35 56.21,25.35 C47.- 56.21,30.3 C46.- | v35.13,34.57 35.13,35.13 C22.2 | C6.2 61.79,14.08 v62.1,13.77 | C33.2 v23.29,25.22 | C20.2 48.51,41.2 v47.85,41.2 | C2.2 24.59,40.56 JTAG.2 | C5.1 v47.95,26.01 C4.1 | C18.2 50.95,45.47 v50.85,45.57 | v38.96,31.88 40.72,31.06 C38.-
  Bottom 0.61: v7.19,42.44 7.21,42.47
  Bottom 0.635: C29.2 29.49,27.81 29.39,27.91 | C38.- 40.69,31.09
  other vias: 30.94,29.46 49.76,35.05 6.58,38.3 51.77,18.29 25.65,35.79 1.27,14.3 1.3,12.75 37.92,5.84 40.46,5.82 48.34,2.54 44.27,5.84 56.06,23.77 60.48,23.77 54.18,38.02 56.77,37.97 54.05,40.77 18.64,11.2 36.22,26.85 31.22,27.81 19.68,14.78 22.94,3.56 62.43,46.13 11.43,38.23 64.85,49.56 51.1,21.74
  pour Top (isolate 0.305, rank 2, no thermals): 1.27,52.7 64.07,52.7 arc-45 64.18,52.66 65.41,51.44 65.41,40.47 67.91,37.97 68.45,37.97 68.45,34.92 69.85,34.92 69.85,33.66 67.82,33.66 67.82,35.69 60.83,35.69 60.81,34.04 62.36,34.04 64.26,32 64.26,31.88 67.06,31.88 67.31,31.62 69.98,31.65 69.98,30.73 68.07,30.73 68.07,28.19 67.94,5.52 arc-45 67.9,5.42 65.53,3.05 65.53,1.33 arc-45 65.49,1.23 64.9,0.64 1.14,0.64 arc-90 0.64,1.14 0.64,52.07 arc-90
  pour Bottom (isolate 0.305, rank 2, no thermals): 0.64,52.7 64.14,52.7 65.41,51.44 65.41,38.86 64.14,37.59 64.14,34.29 67.94,30.48 67.94,5.59 65.53,3.17 65.53,0.51 0.64,0.51
HD_CS  (via drill 0.46)
  Top 0.203: IC5.39 52.57,39.73 49.17,39.73 48.23,38.81 48.23,29.64 45.95,27.33 45.95,22.73 45.72,22.48 v44.96,21.72 | U1.39 33.34,17.7 32.89,17.25 v32.89,16.28 32.64,15.62 RR2.3 | v40.72,13.46 41.73,12.45 44.2,12.45 46.99,15.24 46.99,19.68 46.48,20.19 v46.48,20.32
  Bottom 0.203: v32.89,16.28 34.47,14.71 35.15,14.71 35.84,14.02 40.16,14.02 v40.72,13.46 | v44.96,21.72 45.09,21.72 v46.48,20.32
HD_D2  (via drill 0.46)
  Top 0.203: RR1.2 37.57,15.36 37.57,17.02 v38.1,17.75 | IC5.43 52.53,37.29 51.99,37.29 51.46,36.75 51.46,35.28 49.86,33.66 49.86,24.66 48.26,23.06 48.26,22.35 v47.65,21.69
  Bottom 0.203: v38.1,17.75 38.1,17.22 38.63,16.69 44.02,16.69 44.48,16.23 45.9,16.23 47.7,18.03 47.7,21.13 v47.65,21.69
HD_IRQ  (via drill 0.46)
  Top 0.203: IC5.2 54.2,36.61 54.2,35.87 51.26,32.92 51.26,23.42 50.29,22.45 50.29,21.13 50.88,20.55 54.81,20.55 55.4,19.96 55.37,10.67 55.65,10.39 v55.65,8.36 | RR2.4 31.69,15.26 31.19,15.27 v31.19,15.37
  Top 0.254: U1.24 24.07,23.2 23.9,23.04 23.9,22.1 25.53,20.47 v25.53,19.18
  Bottom 0.203: v55.65,8.36 55.6,8.33 49.12,8.33 48.03,9.42 38.61,9.42 36.55,11.51 34.72,11.51 34.16,12.06 34.16,12.83 33.53,13.46 33.1,13.46 v31.19,15.37 28.78,17.78 27.05,17.78 25.65,19.18 v25.53,19.18
HD_LFC  (via drill 0.46)
  Top 0.203: IC5.36 52.55,41.5 50.77,41.5 50.65,41.38 50.11,41.38 47.78,39.04 47.78,30.56 v47.02,29.82
  Bottom 0.203: R9.2 30,32.99 30.05,33.05 35.81,33.05 35.99,32.87 39.98,32.87 40.28,32.56 41.53,32.56 44.27,29.82 v47.02,29.82 47.78,29.82 48.11,29.49 R8.2
HD_RESET  (via drill 0.46)
  Top 0.203: v21.97,23.52 21.76,23.73 RR3.6 | IC5.34 51.32,42.73 50.88,43.18 48.39,43.18 48.01,43.56 v48.01,44.68
  Top 0.254: U1.28 27.84,22.53 27.58,22.78 v27.46,22.78
  Bottom 0.203: v27.46,22.78 22.71,22.78 21.97,23.5 v21.97,23.52 21.61,23.52 20.19,24.89 20.19,25.58 18.72,27.05 18.72,39.47 16.31,41.88 16.31,42.7 18.19,44.58 26.75,44.58 28.42,42.9 40.49,42.9 41.58,43.99 46.76,43.99 47.45,44.68 v48.01,44.68
HD_SHDN  (via drill 0.46)
  Top 0.203: IC5.23 58.4,44.05 58.4,45.03 58.75,45.39 60.25,45.39 v60.76,44.91 | v28.83,22.78 U1.30
  Top 0.254: RR3.7 21.58,24.53 v21.87,24.82 | v61.54,20.45 61.72,20.62 61.72,24.13 62.23,24.64 62.23,31.47 62.1,31.65 v62.03,31.7
  Bottom 0.203: v60.76,44.91 63.37,44.91 63.96,44.32 63.96,40.23 62.61,38.89 62.61,35.43 61.47,34.29 61.47,32.64 62.03,32.08 v62.03,31.7 | v21.87,24.82 23.04,23.65 27.96,23.65 v28.83,22.78 29.29,22.33 33.88,22.33 35.69,24.13 40.66,24.13 41.88,22.91 48.34,22.91 50.32,20.93 61.06,20.93 v61.54,20.45
ID  (via drill 0.46)
  Top 0.254: v9.6,21.57 9.58,22.58 9.25,22.91 8.32,22.92 J2.2
  Bottom 0.254: v9.6,21.57 9.5,21.84 8.76,21.84 8.21,22.39 RR4.5
INT1  (via drill 0.46)
  Top 0.254: v15.98,22.68 15.98,22.53 16.89,21.61 16.89,19.3 16.6,19.01 IC4.14
  Bottom 0.254: v15.98,22.68 15.95,22.68 16.2,22.43 18.49,22.43 19.3,23.24 19.3,25.65 18.14,26.82 18.14,39.27 15.8,41.6 15.8,42.98 17.96,45.14 27,45.14 28.68,43.46 40.11,43.46 41.22,44.58 46.38,44.58 49.81,48.01 53.09,48.01 DIGITAL_1.4
INT13  (via drill 0.46)
  Top 0.203: U1.55 42.63,24.7 43.31,24.03 43.31,22.35 v42.95,22 | IC4.7 22.14,19.01 23.75,17.4 26.42,17.4 27.81,18.8 v27.81,19.28
  Bottom 0.203: v42.95,22 42.95,20.52 41.35,18.92 39.37,18.92 38.89,19.41 36.17,19.41 35.64,19.94 28.47,19.94 v27.81,19.28
IOREF  (via drill 0.46)
  Top 0.203: C41.1 13.5,15.71
  Top 0.305: IC4.19 13.55,15.76 C41.1 13.34,15.75 12.45,15.75 11.56,14.86 11.56,13.08 12.95,11.68 12.95,11.56 13.72,10.79 v13.97,10.79
  Bottom 0.305: v13.97,10.79 14.73,10.03 14.73,6.86 16.38,5.21 16.38,2.03 17.53,0.89 29.59,0.89 30.48,1.78 POWER.7 30.48,3.43 SEL.2
MEXTINT  (via drill 0.46)
  Top 0.203: U1.54 41.94,24.2 v42.37,23.77
  Bottom 0.203: v42.37,23.77 42.75,23.39 48.34,23.39 49.02,24.08 49.02,29.54 48.11,30.45 48.11,34.37 MACB.8
MISO  (via drill 0.46)
  Top 0.203: IC4.16 18.03,17.71 v18.11,17.63
  Bottom 0.203: ICSP.1 61.57,28.42 61.57,24.05 64.39,21.23 64.39,13.06 58.8,7.47 49.2,7.47 47.7,8.97 38.23,8.97 36.27,10.92 32.77,10.92 30.99,12.7 30.99,13.72 28.07,16.64 26.36,16.64 25.78,17.22 18.52,17.22 v18.11,17.63
MISO3  (via drill 0.46)
  Top 0.203: v39.37,4.57 38.86,5.08 38.86,7.49 35.31,11.05 34.16,11.05 v33.27,11.81 | v57.15,4.45 57.4,4.57 60.83,4.57 61.98,5.71 61.98,12.06 62.36,12.45 63.5,12.45 J1.7 | v19.68,19.43 19.68,18.41 20.45,17.65 21.23,17.65 IC4.5 22.12,17.71 23.34,16.48 26.99,16.48 30.35,19.85 30.35,20.94 U1.33
  Bottom 0.203: v39.37,4.57 39.37,4.83 56.77,4.83 v57.15,4.45 | v33.27,11.81 33.27,12.06 28.07,17.27 26.54,17.27 25.91,17.91 20.57,17.91 19.68,18.8 v19.68,19.43
MMDC  (via drill 0.46)
  Top 0.254: U1.76 38.84,36.78 v39.65,36.78
  Bottom 0.203: v39.65,36.78 39.78,35.48 41.27,33.86 42.19,33.86 44.55,31.5 45.57,31.5 45.97,31.9 45.97,32.13 MACB.14
MMDIO  (via drill 0.46)
  Top 0.203: v38,34.62 38,34.9 38.35,35.26 38.35,36.44 U1.77
  Bottom 0.203: MACB.12 47.17,32.77 47.17,32.03 46.1,30.96 44.4,30.96 41.94,33.43 40.95,33.43 39.75,34.62 v38,34.62
MOSI  (via drill 0.46)
  Top 0.203: IC4.17 17.23,17.06 v18.26,16.03
  Bottom 0.203: v18.26,16.03 18.77,16.54 25.65,16.54 26.19,16 28.07,16 30.48,13.59 30.48,12.39 32.46,10.41 35.92,10.41 37.82,8.51 47.32,8.51 48.82,7.01 59.11,7.01 64.92,12.83 64.92,21.49 62.03,24.38 62.03,28.07 63.2,29.23 64.87,29.23 ICSP.4
MOSI3  (via drill 0.46)
  Top 0.203: U1.36 31.83,20.94 31.83,19.89 31.62,19.68 30.91,19.68 28.45,17.22 28.45,17.14 27.33,16.03 23.14,16.03 22.15,17.02 21.46,17.02 IC4.4 20.02,17.06 18.92,18.16 18.92,18.92 v18.41,19.43 | v10.92,11.56 10.79,11.68 10.79,20.32 v11.3,20.83 | J1.3 63.5,16.89 62.36,16.89 62.23,16.76 59.94,16.76 58.29,15.11 58.29,13.84 v59.94,12.19 | v27.43,13.21 27.81,13.21 31.24,16.64 v31.62,16.64
  Bottom 0.203: v59.94,12.19 53.47,12.19 52.32,13.34 44.32,13.34 43.56,12.57 40.26,12.57 39.27,13.56 35.46,13.56 34.92,14.1 33.66,14.1 32,15.75 32,16.26 v31.62,16.64 | v10.92,11.56 11.38,12.01 23.09,12.01 24.26,13.21 v27.43,13.21 | v11.3,20.83 11.56,21.08 12.95,21.08 14.35,19.68 18.16,19.68 v18.41,19.43
MRX_DV  (via drill 0.46)
  Top 0.254: U1.95 29.34,36.46 29.34,35.26 30,34.59 v30.58,34.59
  Bottom 0.203: MACB.10 47.62,33.58 47.62,31.67 46.43,30.48 44.25,30.48 41.73,32.99 40.62,32.99 40.31,33.3 36.32,33.3 35.99,33.63 31.5,33.63 30.58,34.54 v30.58,34.59
MRX_ER  (via drill 0.46)
  Top 0.254: U1.75 42.11,34.7 v42.09,34.7
  Bottom 0.254: v42.09,34.7 42.27,34.7 44.3,32.66 44.73,32.66 MACB.13
MRXD0  (via drill 0.46)
  Top 0.203: U1.73 39.4,33.7 38.84,34.27 38.84,35.05 39.62,35.84 39.95,35.84 40.89,36.78 v41.66,36.78
  Bottom 0.254: v41.66,36.78 42.09,36.35 42.93,36.35 44.32,34.95 MACB.9
MRXD1  (via drill 0.46)
  Top 0.254: U1.74 39.61,34.2 39.32,34.49 39.32,34.85 39.8,35.33 40.69,35.33 v41,35.64
  Bottom 0.254: v41,35.64 42.57,35.64 44.25,33.96 44.7,33.96 MACB.11
MTX_CLK
  Top 0.254: U1.65 43.88,29.7 45.54,31.37 46.63,31.37 47.27,32 47.27,40.49 46.66,41.1 45.31,41.1 44.98,40.77 MACB.1
MTX_EN
  Top 0.254: U1.66 43.26,30.2 44.04,31.01 44.04,38.1 44.7,38.73 44.96,38.73 MACB.3
MTXD0  (via drill 0.46)
  Top 0.254: U1.70 42.13,32.2 43.54,33.6 43.54,39.34 v43.59,39.4
  Bottom 0.254: v43.59,39.4 43.59,37.95 44.04,37.49 MACB.5
MTXD1  (via drill 0.46)
  Top 0.254: U1.71 41.8,32.7 42.98,33.88 42.98,37.31 v42.67,37.59
  Bottom 0.254: v42.67,37.59 44.12,36.22 MACB.7
N$1
  Top 0.254: R6.1 49.97,15.43 | 49.97,15.43 50.04,15.49 | 49.97,15.43 49.22,15.43 IC3.P$5
N$2  (via drill 0.46)
  Top 0.254: U1.6 26.72,32.21 v27.1,32.59
  Bottom 0.254: v27.1,32.59 27.18,32.51 R9.1
N$3  (via drill 0.46)
  Top 0.203: IC6.2 35.81,43.71 36.27,44.17 36.27,44.88 v38.1,46.71 38.1,46.99
  Bottom 0.203: v38.1,46.71 38.1,47.8 39.12,48.82 DIGITAL_2.2
N$4
  Top 0.254: IC5.19 60.35,42.14 60.48,42.01 C24.1
N$5
  Top 0.203: 13.1,42.46 D1.2 | 13,42.46 12.19,41.66 12.19,41.33 10.9,40.03 10.01,40.03 9.53,40.51 9.53,41.15 10.16,41.78 10.16,42.15
  Top 0.305: 13.1,42.46 13,42.46 | 10.16,42.15 IC2.2
N$6
  Top 0.254: IC5.22 62.08,43.94 C26.1
N$7
  Top 0.508: RA.2 RB.2 15.93,11.58 15.93,10.9 16.4,10.42 IC8.3
N$8  (via drill 0.46)
  Top 0.254: IC1.7 v39.98,41.07
  Bottom 0.254: v39.98,41.07 39.88,40.95 39.75,40.77 39.75,40.02 R3.1
N$9
  Bottom 0.305: 68.58,5.08 74.93,11.43
N$10  (via drill 0.46)
  Top 0.762: IC7.1 v52.15,30.89
  Bottom 0.406: R14.1 R16.2
  Bottom 0.508: R14.1 52.85,30.19 v52.15,30.89
N$17  (via drill 0.46)
  Top 0.508: v15.75,7.26 16.4,7.26 IC8.4
  Bottom 0.508: v15.75,7.26 15.88,7.37 R13.1
N$18
  Top 0.508: IC8.1 19.68,9.78 C39.1 20.12,11.66 D4.C
N$20
  Top 0.254: IC5.27 55.98,45.09 56.21,45.31 C28.1
N$31
  Top 0.254: C30.1 53.34,45.9 54.15,46.71 55.04,46.71 55.4,46.35 55.4,44.05 IC5.28
N$32
  Top 0.203: IC5.41 52.48,38.53 51.79,38.53 51.66,38.66 50.34,38.66 C32.1
N$33  (1 unrouted)
  Top 0.406: 59.82,34.9 59.82,34.92
  Top 0.508: C7.2 L2.2 58.53,34.9 59.82,34.9
N$34
  Top 0.203: IC5.35 52.53,42.09 51.41,42.09 51.21,42.29 R11.1
N$39  (via drill 0.46)
  Top 0.254: v32.56,47.8 32.56,47.07 33.3,46.33 33.3,44.38 IC6.4
  Top 0.305: L9.A 2.29,39.5 2.29,41 2.72,41.43 v3.79,41.43
  Bottom 0.254: v3.79,41.43 3.79,41.45 9.2,46.86 15.57,46.86 16.66,47.95 32.41,47.95 v32.56,47.8
N$40
  Top 0.508: IC8.6 19.48,7.26 C39.2 23.08,7.9
  pour Top (isolate 0.305, no thermals): 18.29,7.75 19.18,7.77 19.68,8.38 21.08,8.38 21.34,8.64 33.02,8.64 33.66,8 33.66,5.84 32.51,4.7 25.78,4.7 23.75,6.73 18.29,6.73
N$46
  Bottom 0.305: R7.1 7.62,44.32 5.54,42.32 5.54,41.68 3.25,39.4 3.25,28.32 1.98,27.05 1.98,15.39 4.78,12.6 22.84,12.6 24.08,13.84 26.67,13.84 26.92,14.1 27.81,14.1 28.45,13.46 28.45,11.56 31.24,8.76 33.93,8.76 35.79,6.91 46.18,6.91 47.68,5.41 61.27,5.41 63.5,3.17 ANALOG_IN.6
N$49  (via drill 0.46)
  Top 0.305: D1.1 12.87,44.38 12.75,44.5 12.75,45.92 v12.8,45.97
  Bottom 0.305: v12.8,45.97 11.18,45.97 9.54,44.34 R7.2
N$52  (via drill 0.46)
  Top 0.61: LINK.C v5.82,37.06
  Bottom 0.254: v5.82,37.06 6.95,37.06 RR5.8
N$53  (via drill 0.46)
  Top 0.61: ERROR.C v5.77,34.67
  Bottom 0.254: RR5.7 6.37,35.27 v5.77,34.67
N$54  (via drill 0.46)
  Top 0.61: DATA.C v5.74,32.26
  Bottom 0.254: v5.74,32.26 5.74,32.94 7.26,34.47 7.93,34.47 RR5.6
N$55  (via drill 0.46)
  Top 0.305: L9.C v5.82,39.5
  Bottom 0.305: v5.82,39.5 R12.1
N$56  (via drill 0.46)
  Top 0.203: U1.100 26.34,36.45 25.93,36.85 18.8,36.85 18.34,37.31 18.34,38.43 17.27,39.5 15.49,39.5 14.76,38.76 14.76,37.74 14.17,37.16 v10.72,37.16 10.74,37.13
  Bottom 0.254: v10.72,37.16 10.37,37.16 RR5.1
N$57  (via drill 0.46)
  Top 0.254: U1.1 24.61,34.7 24.38,34.92 18.29,34.92 17.91,34.54 14.4,34.54 13.69,35.23 v10.82,35.23
  Bottom 0.254: v10.82,35.23 9.33,35.23 RR5.2
N$58
  Top 0.305: IC5.4 55.38,34.78 C7.1
N$59
  Top 0.508: X1.1 X4.1 65.53,32.64 arc-90 64.01,33.91 arc90 62.51,34.9 C48(EXL1).1
N$60  (via drill 0.46)
  Top 0.254: U1.2 23.58,34.2 23.5,34.29 22.23,34.29 22.14,34.2 18.53,34.2 18.06,33.73 18.06,32.59 17.45,31.98 13.41,31.98 12.09,33.3 v10.74,33.3
  Bottom 0.254: v10.74,33.3 10.31,33.76 10.31,34.21 10.05,34.47 RR5.3
N$61
  Top 0.254: J3.1 40.64,11.94 39.29,13.28 39.29,15.54 40.23,16.48 40.23,18.09 39.24,19.07 37.19,19.07 36.35,19.91 U1.45
  Bottom 0.762: R15.2 45.57,11.56 45.92,11.91 J3.1
RD+  (via drill 0.46)
  Top 0.254: U1.49 38.34,19.93 38.63,19.63 39.67,19.63 v40.34,20.3
  Bottom 0.203: v40.34,20.3 40.31,20.32 36.88,20.32 36.32,20.88 14.76,20.88 12.16,23.48 RR4.3
RD-  (via drill 0.46)
  Top 0.203: v38.91,22.63 38.89,22.61 38.46,22.61 37.84,21.99 U1.48
  Bottom 0.203: 36.37,21.89 35.79,21.31 15.11,21.31 12.98,23.44 12.98,23.93 11.83,25.08 RR4.1
  Bottom 0.254: 36.37,21.89 36.37,23.22 36.8,23.65 38.51,23.65 38.91,23.24 v38.91,22.63
RESET  (via drill 0.46)  (1 unrouted)
  Top 0.305: v35,9.12 35,4.52 POWER.6 | IC2.3 10.47,44.51 | v10.49,40.84 10.74,40.84 11.56,41.66 11.56,43.69 10.41,44.83
  Top 0.61: RESET.3 RESET.4 10.47,47.56 IC2.3
  Bottom 0.305: ICSP.5 65.99,23.04 65.99,12.32 59.69,6.02 48.01,6.02 46.51,7.52 36.63,7.52 35.03,9.12 v35,9.12 34.72,9.4 31.75,9.4 29.21,11.94 29.21,13.46 27.94,14.73 26.67,14.73 26.47,14.53 23.88,14.53 22.48,13.13 5.28,13.13 2.64,15.77 2.64,26.82 4.01,28.19 4.01,39.14 5.71,40.84 v10.49,40.84 10.54,40.89 | 10.54,40.89 10.58,40.93 | R5.2 9.54,41.9 10.54,40.89
RID  (via drill 0.46)
  Top 0.203: v41.91,21.21 41.91,22.23 41.4,22.73 40.62,22.73 U1.51
  Bottom 0.203: RR4.4 12.17,22.68 14.43,20.42 35.94,20.45 36.52,19.86 39.32,19.86 39.75,19.43 41.02,19.43 41.91,20.32 v41.91,21.21
RXD
  Top 0.254: FTDI.4 17.96,29.13 17.96,27.53 17.35,26.92 15.54,26.92 14.07,25.45 14.07,20.47 14.23,20.31 IC4.12
RXD3
  Top 0.203: U1.26 26.85,20.27 26.86,20.26 26.42,19.81 26.42,18.8 25.93,18.31 24.18,18.31 22.18,20.31 IC4.9
SCK  (via drill 0.46)
  Top 0.203: v17.37,14.66 17.37,15.77 16.74,16.41 IC4.18
  Bottom 0.203: v17.37,14.66 18.26,14.66 19.56,15.95 25.38,15.95 25.96,15.37 28.07,15.37 29.97,13.46 29.97,12.06 32.08,9.96 35.59,9.96 37.52,8.03 46.97,8.03 48.46,6.53 59.36,6.53 65.48,12.65 65.48,21.77 62.48,24.77 62.48,26.8 ICSP.3
SCK3  (via drill 0.46)
  Top 0.203: U1.37 32.34,19.64 31.89,19.19 31.51,19.19 v30.23,17.78 27.86,15.54 22.96,15.54 22.1,16.41 IC4.3 | J1.5 59.73,14.65 v59.18,14.61
  Bottom 0.203: v59.18,14.61 56.77,14.61 55.5,13.34 54.1,13.34 52.83,14.61 43.43,14.61 42.67,15.37 37.34,15.37 35.56,17.14 35.56,17.53 35.05,18.03 33.35,18.03 32.83,17.51 31.13,17.51 30.86,17.78 v30.23,17.78
SD_CS  (via drill 0.46)
  Top 0.203: 8.89,37.47 10.41,38.99 10.97,38.99 11.02,39.04 13.54,39.04 | 13.84,14.22 14.48,15.11 IC4.20
  Top 0.254: v8.89,29.08 8.89,37.47 | v13.21,14.22 13.84,14.22 | 13.54,39.04 14.86,40.39 14.86,40.64 v15.11,40.89
  Bottom 0.203: v8.89,29.08 6.22,29.08 4.83,27.69 4.32,27.69 3.3,26.67 | 3.3,24.89 3.3,16.26 5.46,13.97 12.95,13.97 v13.21,14.22
  Bottom 0.254: v15.11,40.89 15.11,41.02 15.24,41.15 15.24,43.18 17.78,45.72 27.3,45.72 29.03,43.99 30.4,43.99 30.48,44.07 39.75,44.07 40.89,45.21 45.97,45.21 49.4,48.64 52.83,48.64 53.34,49.15 DIGITAL_1.5 | 3.3,24.89 3.3,26.67
SD_CS3  (via drill 0.46)
  Top 0.203: v61.34,17.78 61.72,17.91 63.12,17.91 J1.2 | v32.38,18.41 32.13,18.41 28.77,15.05 22.16,15.05 22.1,15.11 IC4.1
  Bottom 0.203: v61.34,17.78 58.17,17.78 55.88,15.62 44.2,15.62 43.56,16.26 37.97,16.26 37.26,16.97 37.26,17.98 36.78,18.47 35.51,18.47 35.31,18.67 32.64,18.67 v32.38,18.41
SPI1_MISO  (via drill 0.46)
  Top 0.203: IC5.1 53.59,36.62 53.59,35.99 50.8,33.2 50.8,23.88 49.78,22.86 49.78,19.94 IC3.P$8 51.51,19.3 v51.84,19.63 | U1.42 34.85,20.95 34.85,19.2 v36.42,17.63 35.88,17.09 RR1.4 | v54.51,14.38 54.51,19.02 v54.08,19.51
  Bottom 0.203: v54.08,19.51 52.02,19.46 v51.84,19.63 | v54.51,14.38 53.82,15.06 43.87,15.06 43.13,15.8 37.57,15.8 36.42,16.94 v36.42,17.63
SPI1_MOSI  (via drill 0.46)
  Top 0.203: U1.41 34.34,18.64 34.95,18.03 v34.95,16.28 34.95,16.14 RR2.1 | IC5.40 49.3,39.13 48.72,38.61 48.72,29.21 46.43,26.92 46.43,22.43 45.85,21.84 45.85,21.08 45.15,20.38 | v42.27,14.28 42.27,13.61 42.98,12.9 43.89,12.9 46.48,15.49 46.48,19.05 45.15,20.38 | IC3.P$1 41.78,19.43 43.31,19.43 43.94,20.07 44.83,20.07 45.15,20.38
  Bottom 0.203: v34.95,16.28 35.08,16.64 36.78,14.94 41.63,14.94 v42.27,14.28
SPI1_SCK  (via drill 0.46)
  Top 0.203: U1.40 33.84,17.84 v33.91,17.02 33.91,16 33.55,15.64 RR2.2 | IC5.44 52.58,35.64 50.34,33.4 50.34,24.26 48.87,22.78 v48.87,21.11 | v56.97,19.89 56.97,14.55 v56.95,13.26 | IC3.P$2 43.43,18.03 43.94,18.54 43.94,19.05 44.32,19.43 45.34,19.43 45.97,18.8 45.97,16 43.74,13.77 v43.48,13.77
  Bottom 0.203: v33.91,17.02 33.91,16.03 34.65,15.29 35.61,15.29 36.4,14.5 40.84,14.5 42.14,13.21 43.16,13.21 43.46,13.51 v43.48,13.77 43.69,13.97 52.58,13.97 53.82,12.75 56.39,12.75 56.95,13.31 v56.95,13.26 | v48.87,21.11 48.92,21.11 49.58,20.45 56.41,20.45 v56.97,19.89
SS  (via drill 0.46)
  Top 0.254: 15.62,18.34 IC4.15 14.28,18.36 14.22,18.41 13.03,18.41 12.22,19.23 12.22,27.1 12.62,27.51 v12.62,28.12
  Bottom 0.254: v12.62,28.12 12.75,28.25 12.75,41.71 13.66,42.62 13.66,43.94 17.04,47.32 31.45,47.32 32.08,46.69 34.11,46.69 36.58,49.15 DIGITAL_2.3
SS3
  Top 0.203: U1.25 26,22.7 26.92,23.62 29.21,23.62 29.79,23.04 29.79,22.3 29.34,21.84 U1.31 29.34,19.48 26.8,16.94 23.55,16.94 22.13,18.36 IC4.6
TCK
  Top 0.254: JTAG.1 25.6,43.31 29.54,43.31 31.5,41.35 31.5,38.71 31.85,38.35 31.85,36.41 U1.90
TDI
  Top 0.254: JTAG.9 19.3,42.55 18.8,42.04 18.8,40.95 19.53,40.21 25.17,40.21 26.24,41.27 26.49,41.27 27.46,42.24 29.11,42.24 30.43,40.92 30.43,38.28 30.84,37.87 U1.92
TDO  (via drill 0.46)
  Top 0.254: U1.91 31.34,38.12 30.96,38.51 30.96,41.15 29.34,42.77 26.77,42.77 v26.31,42.32
  Bottom 0.203: JTAG.3 23.57,43.2 23.88,43.51 25.78,43.51 26.29,43 26.29,42.34 v26.31,42.32
TMS
  Top 0.254: JTAG.5 22.35,43.48 22.68,43.81 29.77,43.81 32,41.58 32,38.96 32.33,38.63 U1.89
TXD
  Top 0.254: FTDI.5 15.93,28.19 13.54,25.81 13.54,20.07 13.95,19.66 IC4.13
TXD3
  Top 0.203: U1.27 27.33,20.94 27.33,20.03 26.9,19.6 26.9,18.59 26.16,17.86 23.98,17.86 22.18,19.66 IC4.8
VBUS  (via drill 0.46)
  Top 0.254: v35.41,22.5 36.4,22.5 36.83,21.89 36.83,20.94 U1.46 | D3.A arc-45 10.76,27.25 9.65,27.25 9.09,26.69 arc45 v9.07,26.64 v9.06,26.64 arc45 9.02,26.53 9.02,25.83 8.53,25.34 arc-45 8.42,25.3 J2.5
  Bottom 0.305: v35.41,22.5 34.72,21.82 15.47,21.82 13.84,23.44 13.84,24.21 12.17,25.88 9.89,25.88 arc-45 9.79,25.93 v9.07,26.64
VCC  (via drill 0.46)
  Top 0.406: v26.34,2.01 26.34,1.63 27.13,0.84 44.02,0.84 POWER.1
  Top 0.635: v17.91,5.71 17.53,5.21
  Bottom 0.762: R13.2 18.16,5.97 v17.91,5.71 17.78,5.59 C43.+ 17.8,2.41 18.47,1.75 26.04,1.78 26.26,2.01 v26.34,2.01 26.34,3.86 26.67,4.19 26.67,5.46 27.81,6.6 D2.C
  pour Top (isolate 0.305, no thermals): 14.22,8.89 17.14,8.89 17.55,8.38 17.48,6.1 18.29,6.1 18.29,4.7 18.16,4.57 16.38,4.57 14.22,6.65
X1-40  (via drill 0.46)
  Top 0.203: IC5.24 57.81,44.01 57.81,43.08 v58.12,42.7
  Bottom 0.254: 58.34,42.93 v58.12,42.7 58.76,43.34 C9.1 Y1.1 59.05,45.59 60.45,46.99 C8.2
X2-40  (via drill 0.46)
  Top 0.203: IC5.25 57.2,44.02 57.2,43.1 v56.82,42.72
  Bottom 0.305: C10.2 57.06,46.88 Y1.3 57.02,46.74 56.39,46.74 56.01,46.35 56.01,44.58 56.64,43.94 C9.2 56.82,43.94 v56.82,42.72
XIN0
  Top 0.254: U1.85 34.34,37.95 35,38.61 35,39.59 Q1.1
XIN1
  Top 0.254: Q2.1 29.72,39.61 29.72,38.23 30.34,37.6 U1.93
XIN32  (via drill 0.46)
  Top 0.254: U1.63 41.64,28.7 arc-45 41.75,28.66 v43.23,27.18 43.36,27.05
  Bottom 0.305: 44.76,25.73 43.74,25.73 43.56,25.91 43.56,26.85 v43.23,27.18
  Bottom 0.406: Q3.P$2 arc45 44.91,25.58 44.76,25.73
  Bottom 0.508: 44.91,25.58 46.13,25.58 C4.2
XOUT0
  Top 0.254: U1.86 33.84,37.53 33.1,38.28 33.1,39.56 Q1.3
XOUT1
  Top 0.254: Q2.3 27.71,39.62 27.71,38.28 28.02,37.97 29.23,37.97 29.84,37.37 U1.94
XOUT32  (via drill 0.46)
  Top 0.254: U1.64 42.45,29.2 42.47,29.18 42.49,29.18 43,28.68 v43.26,28.68
  Bottom 0.254: R8.1 C5.2
  Bottom 0.406: v43.26,28.68 46.58,28.68 R8.1
  Bottom 0.508: Q3.P$1 43,28.68 arc46 v43.26,28.68

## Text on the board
tPlace: 9 | 8 | 7 | 6 | 5 | 4 | 3 | 2 | 13 | 12 | 11 | 10 | TX | RX | AREF | GND | DIGITAL | 1 | 1 | 1 | ANALOG IN | RESET | 3.3 | 5 Gnd Vin | 0 1 2 3 4 5
Document: by Designs & Prototypes Engineering | Arduino Wifi Shield | www.arduino.cc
